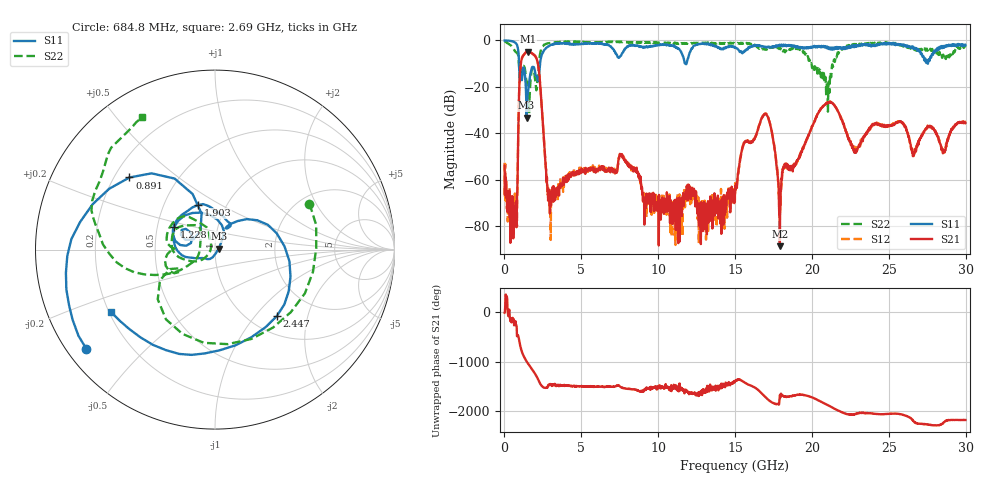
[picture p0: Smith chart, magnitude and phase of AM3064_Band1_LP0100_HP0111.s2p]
# Hz S DB R 50.0
!freq dBS11 angS11 dBS21 angS21 dBS12 angS12 dBS22 angS22
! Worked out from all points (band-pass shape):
!   1600 points, 10 MHz to 29.98 GHz, reference 50 ohm
!   highest |S21| = -4.83 dB at 1.528 GHz (marker M1); lowest = -88.7 dB at 17.91 GHz (marker M2)
!   |S21| within 3 dB of the highest: 1.129 GHz to 2.085 GHz (955.9 MHz wide, 59.5 % of centre)
!   lowest |S11| = -33.4 dB at 1.435 GHz (marker M3), VSWR 1.04, Z = 52.1 + j0.612 ohm
!   |S11| at or under -10 dB: 949.5 MHz to 2.311 GHz (1.362 GHz wide, 83.5 % of centre); 11.76 GHz to 11.84 GHz (82.38 MHz wide, 0.698 % of centre); 27.52436 GHz to 27.54536 GHz (21 MHz wide, 0.0763 % of centre)
!   |S22| runs from -31.8 to -0.4 dB; largest |S21 - S12| = 0.0078
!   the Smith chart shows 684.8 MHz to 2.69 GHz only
!   S11 on the Smith chart (normalised r, x): 684.8 MHz: 0.06, -0.34; 891 MHz: 0.26, +0.34; 1.228 GHz: 0.61, +0.16; 1.903 GHz: 0.74, +0.39; 2.447 GHz: 1.31, -1.31; 2.69 GHz: 0.21, -0.27
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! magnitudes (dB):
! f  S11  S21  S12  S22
! 10 MHz  0.0  -54.0  -52.8  -0.4
! 684.8 MHz  -0.9  -77.0  -66.0  -4.6
! 891 MHz  -4.1  -42.4  -42.7  -6.5
! 1.06 GHz  -13.3  -10.2  -10.2  -10.9
! 1.228 GHz  -11.7  -6.5  -6.4  -11.0
! 1.435 GHz  -33.4  -5.0  -5.0  -17.5
! 1.528 GHz  -22.5  -4.8  -4.8  -22.9
! 1.903 GHz  -11.5  -6.2  -6.2  -12.5
! 2.447 GHz  -5.9  -30.9  -30.8  -2.8
! 2.69 GHz  -3.4  -55.0  -54.8  -1.5
! 3.065 GHz  -1.9  -64.8  -64.8  -1.0
! 5.015 GHz  -1.4  -55.3  -56.0  -0.6
! 7.62 GHz  -6.0  -49.6  -49.5  -0.7
! 10 GHz  -2.0  -71.3  -72.3  -0.9
! 15 GHz  -3.0  -65.9  -61.4  -1.4
! 16.97 GHz  -2.8  -31.7  -31.8  -3.7
! 17.91 GHz  -2.0  -88.7  -76.2  -3.4
! 19.99 GHz  -3.2  -37.5  -37.5  -11.2
! 21.02 GHz  -2.8  -26.8  -26.9  -25.1
! 25 GHz  -1.1  -36.8  -37.1  -1.2
! 26.63 GHz  -3.7  -48.9  -49.8  -3.3
! 29.98 GHz  -1.9  -35.6  -35.3  -2.9
